(* Logix 5000 AddOnInstructionDefinition export ASDG9ETH_Generic_Default_IO; software revision 19.01 *)

ADD_ON_INSTRUCTION ASDG9ETH_Generic_Default_IO   (* revision 1.0 *)
// Simple interface for generic default IO mapping that uses Input Assembly Instance 150 and Output Assembly Instance 100.
VAR_IN_OUT
   I_Data : INT[2]; {required}   // Input data
   O_Data : INT[2]; {required}   // Output data
END_VAR
VAR_INPUT
   FwdRev : BOOL; {access Read Only, required}   // Forward (0) or Reverse (1) direction
   RunStop : BOOL; {access Read Only, required}   // Run (1) or Stop (0)
   FaultReset : BOOL; {required}   // Reset the fault
   FreqPrioritySel : BOOL; {required}   // Frequency priority selection
   CmdPrioritySel : BOOL; {required}   // Command priority selection
   FrequencyCommand : INT; {access Read Only, required}   // Frequency command/reference
END_VAR
VAR_OUTPUT
   Alarm : BOOL; {access Read Only, visible}   // Alarm or Trip
   RunningFwdRev : BOOL; {access Read Only, visible}   // Running forward (0) or reverse (1)
   RunningStopped : BOOL; {access Read Only, visible}   // Running (1) or Stopped (0)
   EStop : BOOL; {access Read Only, visible}   // Emergency stop
   Standby : BOOL; {access Read Only, visible}   // Startup process (0) or Standby (1)
   OutputFrequency : INT; {access Read Only, visible}   // Output/feedback frequency
END_VAR

ROUTINE Logic   (* ladder *)
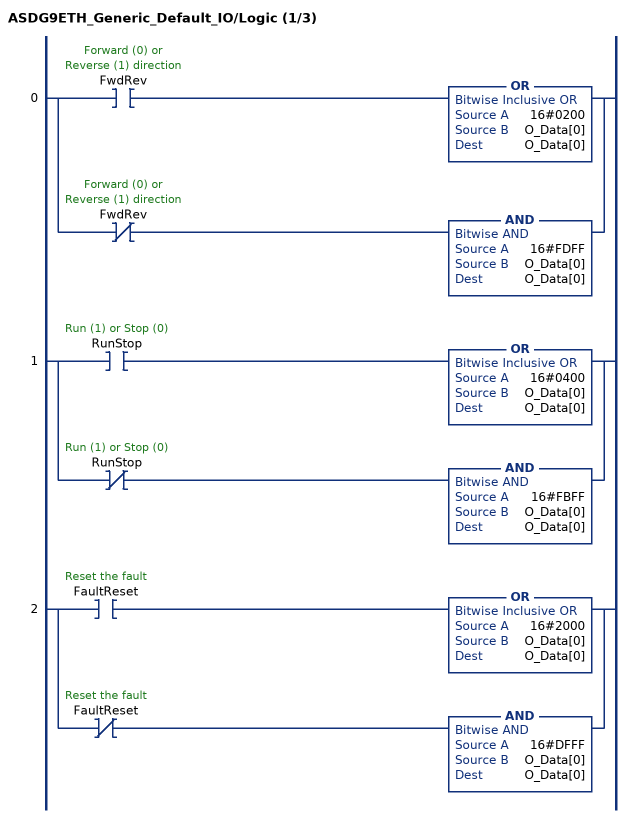
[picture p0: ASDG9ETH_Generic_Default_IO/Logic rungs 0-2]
   0: [XIC(FwdRev) OR(16#0200,O_Data[0],O_Data[0]) ,XIO(FwdRev) AND(16#FDFF,O_Data[0],O_Data[0]) ];
   1: [XIC(RunStop) OR(16#0400,O_Data[0],O_Data[0]) ,XIO(RunStop) AND(16#FBFF,O_Data[0],O_Data[0]) ];
   2: [XIC(FaultReset) OR(16#2000,O_Data[0],O_Data[0]) ,XIO(FaultReset) AND(16#DFFF,O_Data[0],O_Data[0]) ];
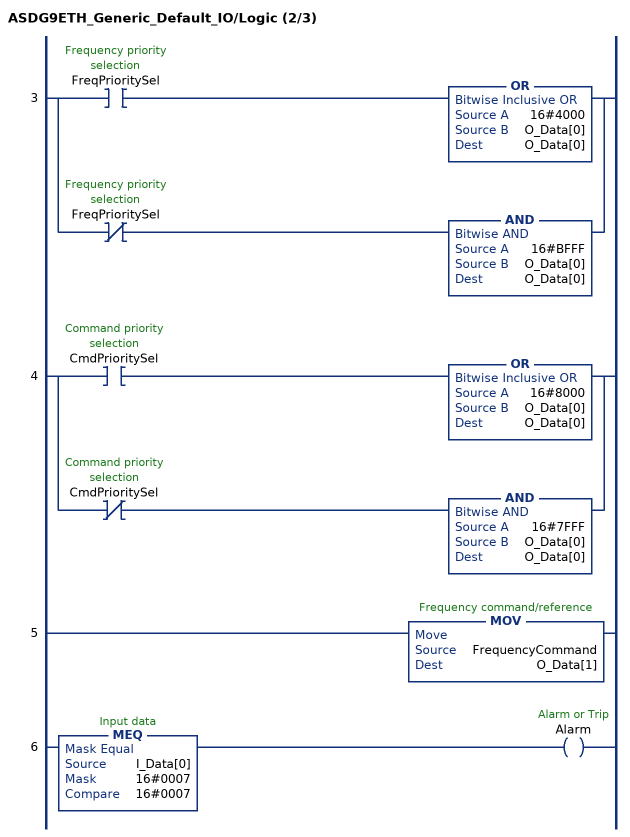
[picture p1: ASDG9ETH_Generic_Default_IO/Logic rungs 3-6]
   3: [XIC(FreqPrioritySel) OR(16#4000,O_Data[0],O_Data[0]) ,XIO(FreqPrioritySel) AND(16#BFFF,O_Data[0],O_Data[0]) ];
   4: [XIC(CmdPrioritySel) OR(16#8000,O_Data[0],O_Data[0]) ,XIO(CmdPrioritySel) AND(16#7FFF,O_Data[0],O_Data[0]) ];
   5: MOV(FrequencyCommand,O_Data[1]);
   6: MEQ(I_Data[0],16#0007,16#0007)OTE(Alarm);
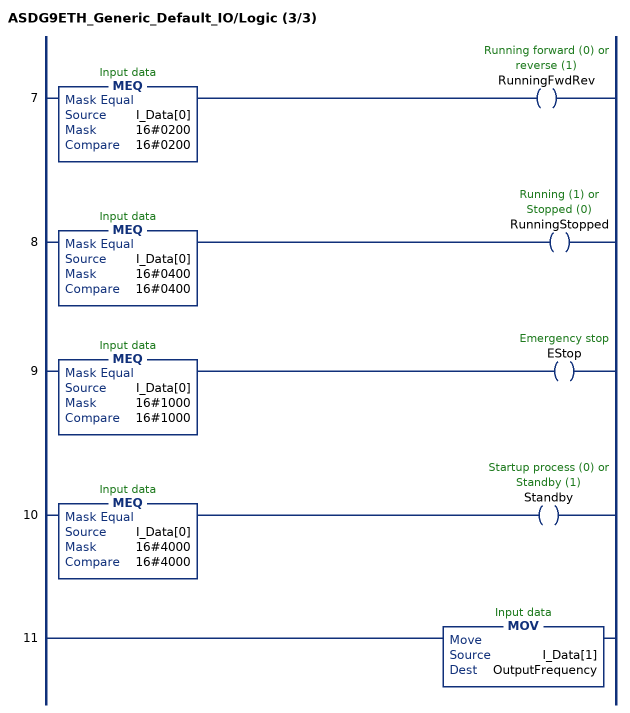
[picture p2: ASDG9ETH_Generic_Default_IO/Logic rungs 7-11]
   7: MEQ(I_Data[0],16#0200,16#0200)OTE(RunningFwdRev);
   8: MEQ(I_Data[0],16#0400,16#0400)OTE(RunningStopped);
   9: MEQ(I_Data[0],16#1000,16#1000)OTE(EStop);
   10: MEQ(I_Data[0],16#4000,16#4000)OTE(Standby);
   11: MOV(I_Data[1],OutputFrequency);
END_ROUTINE
END_ADD_ON_INSTRUCTION
